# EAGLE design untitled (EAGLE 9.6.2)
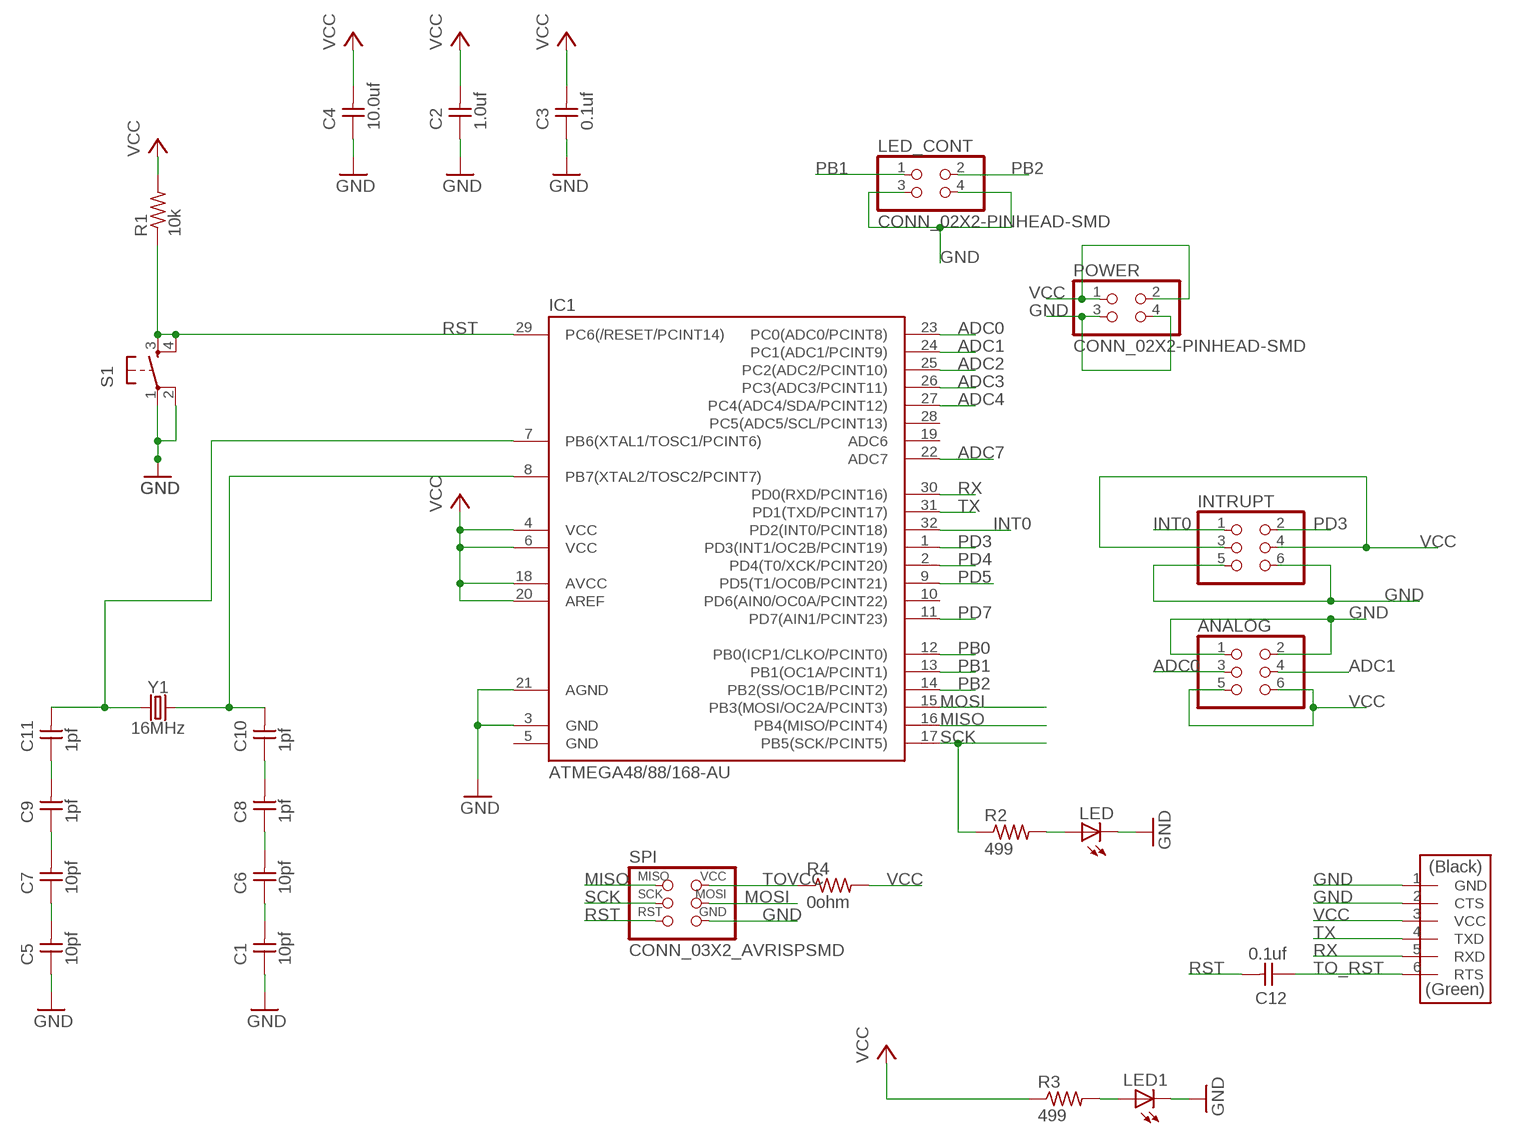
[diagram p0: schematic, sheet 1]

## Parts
ANALOG  CONN_03X2-PINHEAD-SMD  [2X03SMD]
C1  10pf  UNPOLARIZED_CAPACITOR1206  [1206]
C2  1.0uf  UNPOLARIZED_CAPACITOR1206  [1206]
C3  0.1uf  UNPOLARIZED_CAPACITOR1206  [1206]
C4  10.0uf  UNPOLARIZED_CAPACITOR1206  [1206]
C5  10pf  UNPOLARIZED_CAPACITOR1206  [1206]
C6  10pf  UNPOLARIZED_CAPACITOR1206  [1206]
C7  10pf  UNPOLARIZED_CAPACITOR1206  [1206]
C8  1pf  UNPOLARIZED_CAPACITOR1206  [1206]
C9  1pf  UNPOLARIZED_CAPACITOR1206  [1206]
C10  1pf  UNPOLARIZED_CAPACITOR1206  [1206]
C11  1pf  UNPOLARIZED_CAPACITOR1206  [1206]
C12  0.1uf  UNPOLARIZED_CAPACITOR1206  [1206]
IC1  ATMEGA48/88/168-AU  [TQFP32-08]
INTRUPT  CONN_03X2-PINHEAD-SMD  [2X03SMD]
LED  LED1206  [1206]
LED1  LED1206  [1206]
LED_CONT  CONN_02X2-PINHEAD-SMD  [2X02SMD]
POWER  CONN_02X2-PINHEAD-SMD  [2X02SMD]
R1  10k  RESISTOR1206  [1206]
R2  499  RESISTOR1206  [1206]
R3  499  RESISTOR1206  [1206]
R4  0ohm  R1206FAB  [R1206FAB]
S1  6MM_SWITCH6MM_SWITCH  [6MM_SWITCH]
SPI  CONN_03X2_AVRISPSMD  [2X03SMD]
U$1  CONN_06_FTDI-SMD-HEADER  [1X06SMD]
Y1  16MHz  CRYSTAL-16MHZPTH-HC49US  [HC49US]

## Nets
ADC0: ANALOG.3 IC1.23(PC0(ADC0/PCINT8))
ADC1: ANALOG.4 IC1.24(PC1(ADC1/PCINT9))
ADC2: IC1.25(PC2(ADC2/PCINT10))
ADC3: IC1.26(PC3(ADC3/PCINT11))
ADC4: IC1.27(PC4(ADC4/SDA/PCINT12))
ADC7: IC1.22(ADC7)
GND: ANALOG.1 ANALOG.2 C1.1 C2.1 C3.1 C4.1 C5.1 IC1.3(GND) IC1.21(AGND) INTRUPT.5 INTRUPT.6 LED1.2(C) LED.2(C) LED_CONT.3 LED_CONT.4 POWER.3 POWER.4 S1.1(P) S1.2(P1) SPI.6(GND) U$1.1(GND) U$1.2(CTS)
INT0: IC1.32(PD2(INT0/PCINT18)) INTRUPT.1
MISO: IC1.16(PB4(MISO/PCINT4)) SPI.1(MISO)
MOSI: IC1.15(PB3(MOSI/OC2A/PCINT3)) SPI.4(MOSI)
N$1: C11.2 IC1.7(PB6(XTAL1/TOSC1/PCINT6)) Y1.1
N$2: LED1.1(A) R3.2
N$3: C8.2 C10.1
N$4: C9.2 C11.1
N$5: C7.2 C9.1
N$6: C6.2 C8.1
N$7: C10.2 IC1.8(PB7(XTAL2/TOSC2/PCINT7)) Y1.2
N$8: C1.2 C6.1
N$10: C5.2 C7.1
N$23: LED.1(A) R2.2
PB0: IC1.12(PB0(ICP1/CLKO/PCINT0))
PB1: IC1.13(PB1(OC1A/PCINT1)) LED_CONT.1
PB2: IC1.14(PB2(SS/OC1B/PCINT2)) LED_CONT.2
PD3: IC1.1(PD3(INT1/OC2B/PCINT19)) INTRUPT.2
PD4: IC1.2(PD4(T0/XCK/PCINT20))
PD5: IC1.9(PD5(T1/OC0B/PCINT21))
PD7: IC1.11(PD7(AIN1/PCINT23))
RST: C12.2 IC1.29(PC6(/RESET/PCINT14)) R1.1 S1.3(S) S1.4(S1) SPI.5(RST)
RX: IC1.30(PD0(RXD/PCINT16)) U$1.5(RXD)
SCK: IC1.17(PB5(SCK/PCINT5)) R2.1 SPI.3(SCK)
TO_RST: C12.1 U$1.6(RTS)
TOVCC: R4.1 SPI.2(VCC)
TX: IC1.31(PD1(TXD/PCINT17)) U$1.4(TXD)
VCC: ANALOG.5 ANALOG.6 C2.2 C3.2 C4.2 IC1.4(VCC) IC1.6(VCC) IC1.18(AVCC) IC1.20(AREF) INTRUPT.3 INTRUPT.4 POWER.1 POWER.2 R1.2 R3.1 R4.2 U$1.3(VCC)
Unconnected: IC1.10(PD6(AIN0/OC0A/PCINT22)) IC1.19(ADC6) IC1.28(PC5(ADC5/SCL/PCINT13))

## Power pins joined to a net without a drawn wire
GND: IC1.5(GND)

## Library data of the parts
ANALOG INTRUPT = fab:CONN_03X2-PINHEAD-SMD: PIN HEADER
C1-C12 = ng:UNPOLARIZED_CAPACITOR: unpolarized_capacitor
IC1 = atmega8:ATMEGA48/88/168
LED LED1 = ng:LED
LED_CONT POWER = fab:CONN_02X2-PINHEAD-SMD
R1-R3 = ng:RESISTOR
R4 = fab:R: Resistor (US Symbol)
S1 = ng:6MM_SWITCH: OMRON SWITCH
SPI = fab:CONN_03X2_AVRISP
U$1 = fab:CONN_06_FTDI-SMD-HEADER
Y1 = SparkFun-Clocks:CRYSTAL-16MHZ: 16MHz Crystal; PROD_ID: XTAL-08181; SF_ID: COM-00536

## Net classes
0 default: clearance 0.356 mm

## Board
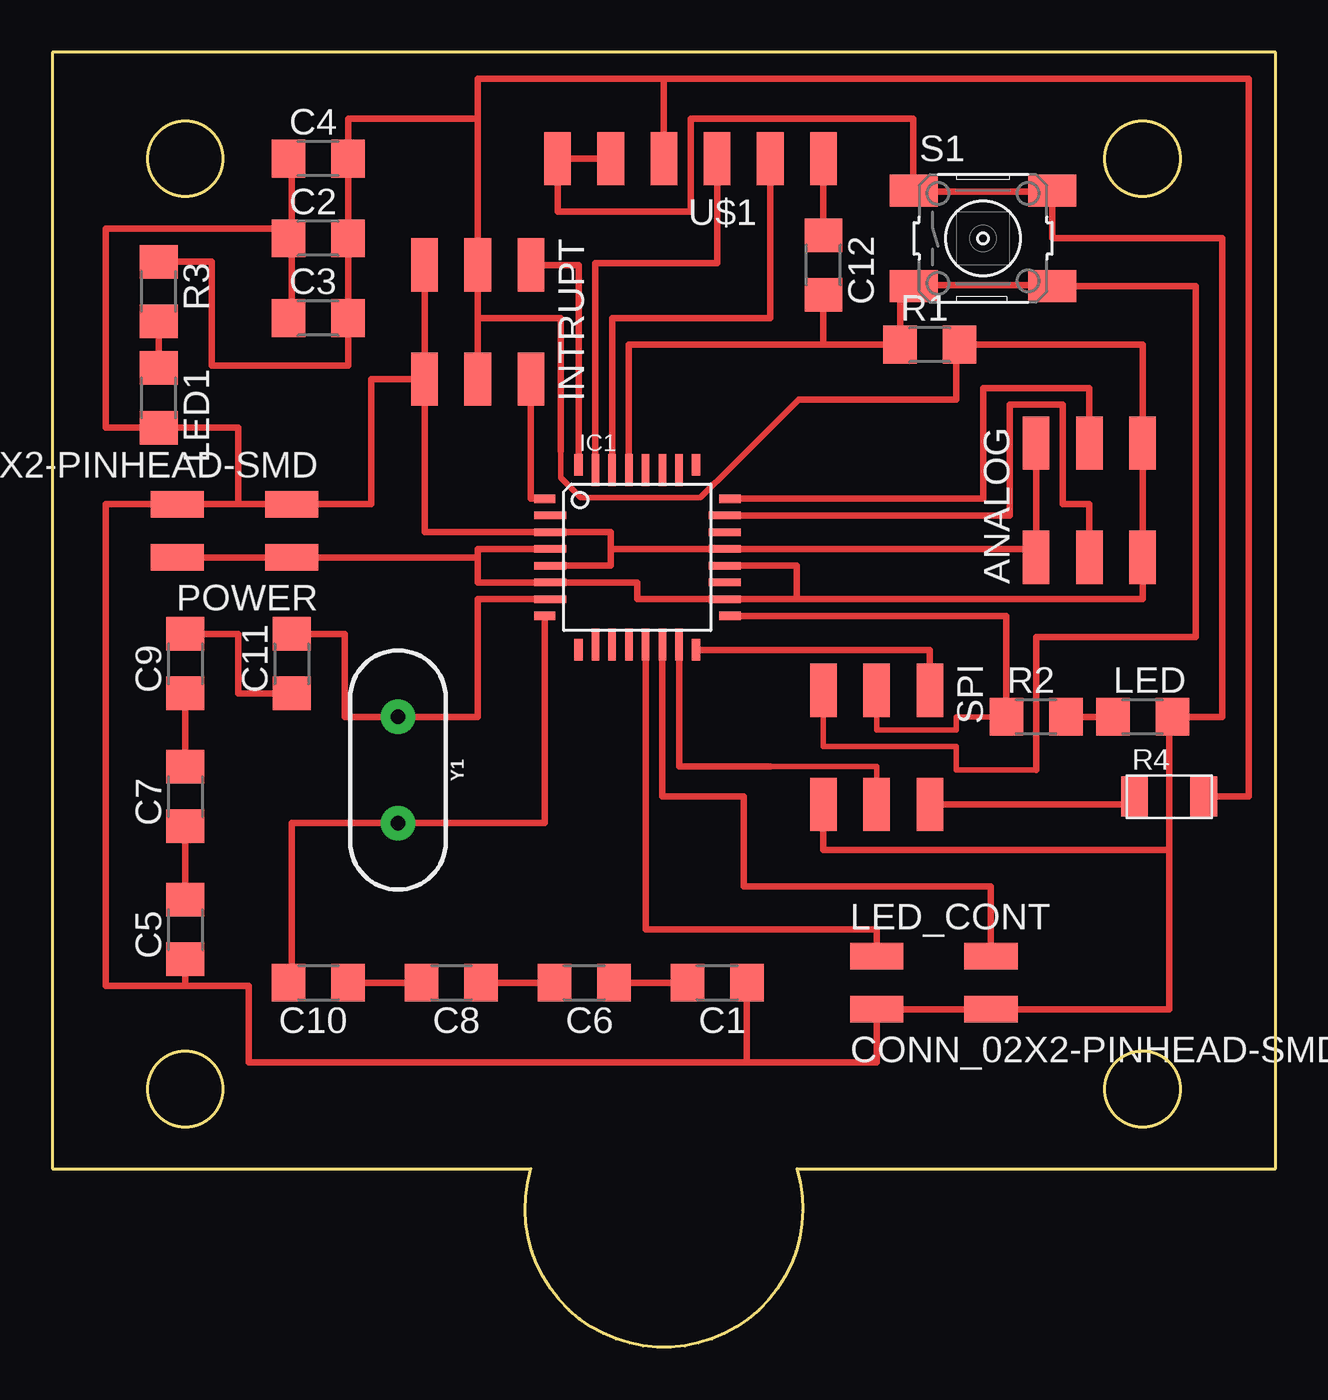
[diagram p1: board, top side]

Size 58.42 x 61.87 mm. Coordinates in mm from the lower left corner, seen from the top.
Outline: 35.56,8.53 arc-213 22.86,8.53 0,8.53 0,61.87 58.42,61.87 58.42,8.53 35.56,8.53
Outline: circle at 6.35,56.79 radius 1.8
Outline: circle at 6.35,12.34 radius 1.8
Outline: circle at 52.07,12.34 radius 1.8
Outline: circle at 52.07,56.79 radius 1.8
Copper layers (1*16): Top 0.035mm / dielectric 1.5mm / Bottom 0.035mm
Design rules "default": minimum track width 6mil, minimum drill 0.35mm, track to track 6mil, track to pad 6mil, pad to pad 6mil, via to via 6mil, smd to smd 6mil, copper to edge 40mil, drill to drill 6mil, minimum pad ring 10mil, minimum via ring 8mil, stop-mask expansion 4mil, vias tented up to drill 0mil, thermal gap 10mil

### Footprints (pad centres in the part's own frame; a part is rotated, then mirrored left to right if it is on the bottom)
2X03SMD = smd 2.54 x 1.27: 1 -2.54,2.54; 2 2.92,2.54; 3 -2.54,0; 4 2.92,0; 5 -2.54,-2.54; 6 2.92,-2.54
1206 = smd 1.6 x 1.803: 1 -1.422,0; 2 1.422,0
TQFP32-08 = smd 1.016 x 0.406: 1 -4.42,2.8; 8 -4.42,-2.8; 17 4.42,-2.8; 24 4.42,2.8 | smd 1.524 x 0.356: 2 -4.166,2; 3 -4.166,1.2; 4 -4.166,0.4; 5 -4.166,-0.4; 6 -4.166,-1.2; 7 -4.166,-2; 18 4.166,-2; 19 4.166,-1.2; 20 4.166,-0.4; 21 4.166,0.4; 22 4.166,1.2; 23 4.166,2 | smd 0.406 x 1.016: 9 -2.8,-4.42; 16 2.8,-4.42; 25 2.8,4.42; 32 -2.8,4.42 | smd 0.356 x 1.524: 10 -2,-4.166; 11 -1.2,-4.166; 12 -0.4,-4.166; 13 0.4,-4.166; 14 1.2,-4.166; 15 2,-4.166; 26 2,4.166; 27 1.2,4.166; 28 0.4,4.166; 29 -0.4,4.166; 30 -1.2,4.166; 31 -2,4.166
2X02SMD = smd 2.54 x 1.27: 1 -2.54,1.27; 2 2.92,1.27; 3 -2.54,-1.27; 4 2.92,-1.27
R1206FAB = smd 1.27 x 1.905: 1 -1.651,0; 2 1.651,0
6MM_SWITCH = smd 2.286 x 1.524: 1 -3.302,2.286; 2 3.302,2.286; 3 -3.302,-2.286; 4 3.302,-2.286
1X06SMD = smd 2.54 x 1.27: 1 0,6.35; 2 0,3.81; 3 0,1.27; 4 0,-1.27; 5 0,-3.81; 6 0,-6.35
HC49US = drill 0.7 pad 1.651: 1 -2.54,0; 2 2.54,0

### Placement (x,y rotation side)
ANALOG  49.53,40.28 90 top
C1  31.75,17.42 180 top
C2  12.7,52.98 0 top
C3  12.7,49.17 0 top
C4  12.7,56.79 0 top
C5  6.35,19.96 90 top
C6  25.4,17.42 180 top
C7  6.35,26.31 90 top
C8  19.05,17.42 180 top
C9  6.35,32.66 90 top
C10  12.7,17.42 180 top
C11  11.43,32.66 90 top
C12  36.83,51.71 270 top
IC1  27.94,37.74 0 top
INTRUPT  20.32,49.17 270 top
LED  52.07,30.12 0 top
LED1  5.08,45.36 270 top
LED_CONT  41.91,17.42 0 top
POWER  8.89,39.01 180 top
R1  41.91,47.9 0 top
R2  46.99,30.12 0 top
R3  5.08,50.44 270 top
R4  53.34,26.31 0 top
S1  44.45,52.98 0 top
SPI  39.37,28.85 270 top
U$1  30.48,56.79 90 top
Y1  16.51,27.58 270 top

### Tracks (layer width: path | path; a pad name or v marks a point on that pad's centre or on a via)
ADC0
  Top 0.305: IC1.23 45.72,39.74 45.72,45.04 48.26,45.04 48.26,40.28 49.53,40.28 ANALOG.3
ADC1
  Top 0.305: ANALOG.4 49.53,45.83 44.45,45.83 44.45,40.54 IC1.24
GND
  Top 0.305: 44.93,16.15 LED_CONT.4 | ANALOG.2 46.99,38.21 | 46.99,38.21 ANALOG.1 | INTRUPT.5 INTRUPT.6 | 11.43,52.98 11.43,49.17 C3.1 | 11.43,52.98 11.43,53.45 | 11.43,53.45 11.43,56.79 C4.1 | 11.43,52.98 C2.1 11.43,53.45 | 8.89,40.28 POWER.3 15.24,40.28 15.24,46.25 INTRUPT.6 | 6.35,17.26 C5.1 | 11.43,53.45 2.54,53.45 2.54,43.93 LED1.2 8.89,43.93 8.89,40.28 | 6.35,17.26 2.54,17.26 2.54,40.28 POWER.4 8.89,40.28 | 33.17,13.61 9.39,13.61 9.39,17.26 6.35,17.26 | 33.17,13.61 39.37,13.61 LED_CONT.3 LED_CONT.4 | 53.34,23.77 53.34,16.15 LED_CONT.4 | 53.34,23.77 53.34,30.12 LED.2 55.88,30.12 55.88,52.98 47.75,52.98 S1.2 47.62,55.2 41.27,55.2 S1.1 41.12,55.36 41.12,58.69 30.48,58.69 30.48,54.25 24.13,54.25 U$1.1 U$1.2 | 53.34,23.77 36.83,23.77 SPI.6 | IC1.5 26.67,37.34 26.67,38.21 | 26.67,38.21 26.67,38.94 IC1.3 17.78,38.94 INTRUPT.6 | C1.1 33.17,13.61 | 26.67,38.21 26.75,38.14 IC1.21 46.91,38.14 46.99,38.21
INT0
  Top 0.305: INTRUPT.1 25.14,51.71 IC1.32
MISO
  Top 0.305: SPI.1 41.91,33.32 IC1.16
MOSI
  Top 0.254: SPI.4 39.37,27.74 34.29,27.74
  Top 0.305: IC1.15 29.94,27.74 34.29,27.74
N$1
  Top 0.305: IC1.7 20.32,35.74 20.32,30.12 Y1.1 13.97,30.12 13.97,34.08 C11.2
N$2
  Top 0.305: R3.2 LED1.1
N$3
  Top 0.305: C8.2 C10.1
N$4
  Top 0.305: C9.2 8.89,34.08 8.89,31.23 C11.1
N$5
  Top 0.305: C9.1 C7.2
N$6
  Top 0.305: C6.2 C8.1
N$7
  Top 0.305: C10.2 11.43,17.42 11.43,25.04 Y1.2 23.52,25.04 IC1.8
N$8
  Top 0.305: C1.2 C6.1
N$10
  Top 0.305: C7.1 C5.2
N$23
  Top 0.305: LED.1 R2.2
PB1
  Top 0.305: IC1.13 28.34,19.96 39.37,19.96 LED_CONT.1
PB2
  Top 0.305: IC1.14 29.14,26.31 33.02,26.31 33.02,22.02 44.83,22.02 LED_CONT.2
PD3
  Top 0.305: IC1.1 22.86,40.54 INTRUPT.2
RST
  Top 0.254: SPI.5 36.83,28.71 43.18,28.71 43.18,27.58 46.99,27.58
  Top 0.305: 36.83,47.9 R1.1 40.49,50.69 S1.3 | 41.12,50.6 S1.3 | S1.3 41.27,50.75 47.62,50.75 S1.4 54.61,50.69 54.61,33.93 46.99,33.93 46.99,27.58 | IC1.29 27.54,47.9 36.83,47.9 | C12.2 36.83,47.9
RX
  Top 0.305: U$1.5 34.29,49.17 26.74,49.17 IC1.30
SCK
  Top 0.254: SPI.3 39.37,29.48 43.18,29.48 43.18,30.12 R2.1
  Top 0.305: R2.1 45.57,34.94 IC1.17
TO_RST
  Top 0.305: U$1.6 C12.1
TOVCC
  Top 0.305: R4.1 51.69,25.93 SPI.2
TX
  Top 0.305: IC1.31 25.94,51.79 31.75,51.79 U$1.4
VCC
  Top 0.254: 24.29,42.82 24.29,41.55 25.24,40.59 30.96,40.59 32.46,42.1
  Top 0.305: 20.32,49.17 INTRUPT.3 20.32,58.69 | 20.32,49.17 INTRUPT.4 | C2.2 C3.2 14.12,46.91 7.62,46.91 7.62,51.86 R3.1 | C2.2 C4.2 14.12,58.69 20.32,58.69 | C2.2 | POWER.2 POWER.1 20.32,37.74 | 24.29,42.82 24.29,49.17 20.32,49.17 | 32.46,42.1 35.64,45.28 43.18,45.28 43.18,47.9 R1.2 52.07,47.9 ANALOG.6 ANALOG.5 52.07,35.74 35.56,35.74 | 35.56,35.74 IC1.18 27.94,35.74 27.94,36.54 IC1.6 20.32,36.54 20.32,37.74 | IC1.20 35.56,37.34 35.56,35.74 | IC1.4 20.32,38.14 20.32,37.74 | 29.21,60.6 57.15,60.6 57.15,26.31 R4.2 | U$1.3 29.21,60.6 | 29.21,60.6 20.32,60.6 20.32,58.69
